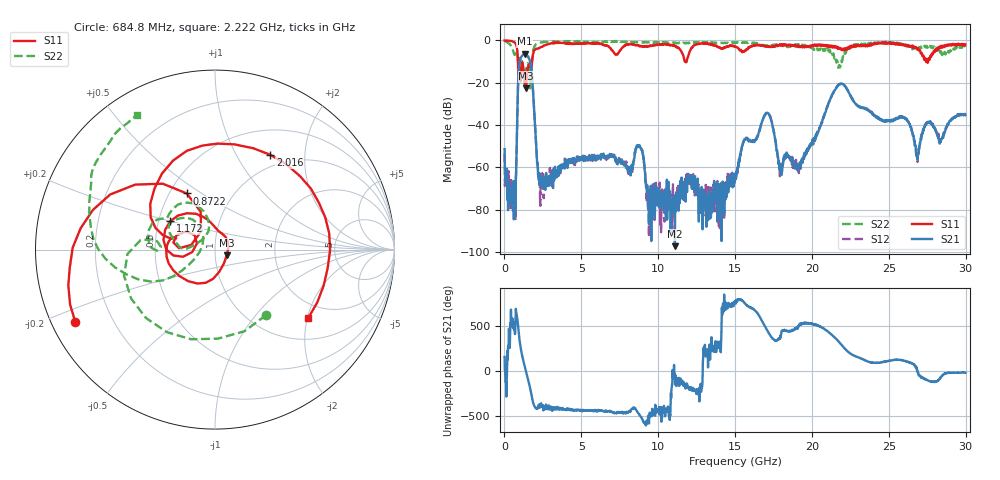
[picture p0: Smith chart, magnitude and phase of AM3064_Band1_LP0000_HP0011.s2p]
# Hz S DB R 50.0
!freq dBS11 angS11 dBS21 angS21 dBS12 angS12 dBS22 angS22
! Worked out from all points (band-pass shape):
!   1600 points, 10 MHz to 29.98 GHz, reference 50 ohm
!   highest |S21| = -6.29 dB at 1.322 GHz (marker M1); lowest = -97.3 dB at 11.09 GHz (marker M2)
!   |S21| within 3 dB of the highest: 1.018 GHz to 1.64 GHz (621.1 MHz wide, 46.7 % of centre)
!   lowest |S11| = -22.7 dB at 1.416 GHz (marker M3), VSWR 1.16, Z = 56.9 - j3.63 ohm
!   |S11| at or under -10 dB: 876.6 MHz to 1.796 GHz (919.2 MHz wide, 68.8 % of centre); 11.74 GHz to 11.84 GHz (105.2 MHz wide, 0.892 % of centre); 27.41115 GHz to 27.43778 GHz (26.63 MHz wide, 0.0971 % of centre)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
!   |S22| runs from -22.7 to -0.2 dB; largest |S21 - S12| = 0.005
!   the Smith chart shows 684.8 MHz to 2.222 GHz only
!   S11 on the Smith chart (normalised r, x): 684.8 MHz: 0.07, -0.24; 872.2 MHz: 0.61, +0.44; 1.172 GHz: 0.58, +0.20; 2.016 GHz: 0.83, +1.40; 2.222 GHz: 1.56, -2.03
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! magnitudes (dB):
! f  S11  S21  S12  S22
! 10 MHz  0.0  -51.4  -53.6  -0.2
! 328.6 MHz  -0.2  -70.2  -76.9  -1.6
! 684.8 MHz  -1.1  -83.4  -74.3  -6.7
! 872.2 MHz  -9.1  -23.3  -23.3  -9.5
! 1.172 GHz  -10.6  -7.1  -7.0  -10.7
! 1.322 GHz  -19.6  -6.3  -6.3  -19.1
! 1.416 GHz  -22.7  -6.6  -6.6  -13.6
! 2.016 GHz  -4.3  -43.6  -43.8  -2.1
! 2.222 GHz  -3.8  -63.4  -62.5  -1.2
! 5.015 GHz  -1.3  -56.1  -55.8  -0.8
! 8.745 GHz  -2.6  -50.1  -49.7  -1.0
! 9.363 GHz  -2.8  -79.9  -71.0  -0.9
! 10 GHz  -2.0  -72.7  -69.0  -0.9
! 11.09 GHz  -2.6  -97.3  -77.7  -1.0
! 15 GHz  -2.9  -66.1  -63.7  -1.3
! 17.05 GHz  -2.9  -34.3  -34.3  -2.7
! 17.95 GHz  -2.3  -61.0  -62.1  -1.9
! 19.99 GHz  -2.9  -48.8  -48.3  -3.4
! 21.85 GHz  -3.6  -20.6  -20.5  -12.1
! 25 GHz  -1.0  -37.8  -38.0  -1.1
! 26.85 GHz  -4.4  -55.2  -53.3  -3.2
! 29.98 GHz  -1.9  -35.3  -35.1  -3.2
